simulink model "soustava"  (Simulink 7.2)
settings: Solver=ode45  StartTime=0.0  StopTime=1  RelTol=1e-3
InitFcn:
  | init_soustava;
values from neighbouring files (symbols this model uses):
  I1 = eye(3)    [init_soustava.m]
  I2 = [(m2/4)*(r2^2 + (h2^2)/3 ) 0 0    [init_soustava.m]
  I3 = [(m3/4)*(r3^2 + (h3^2)/3 ) 0 0    [init_soustava.m]
  m = 1    [smykadlo_init.m]
  m1 = 2    [init_soustava.m]
  m2 = 1    [init_soustava.m]
  m3 = 1    [init_soustava.m]
  r2 = 2    [init_soustava.m]
  r3 = 0.5    [init_soustava.m]
  rr = r3 + r2    (= 2.5)    [init_soustava.m]
undefined symbols (not defined in the file or in its folder): deg, kg, N, rad, s
libraries: mblibv1 x25

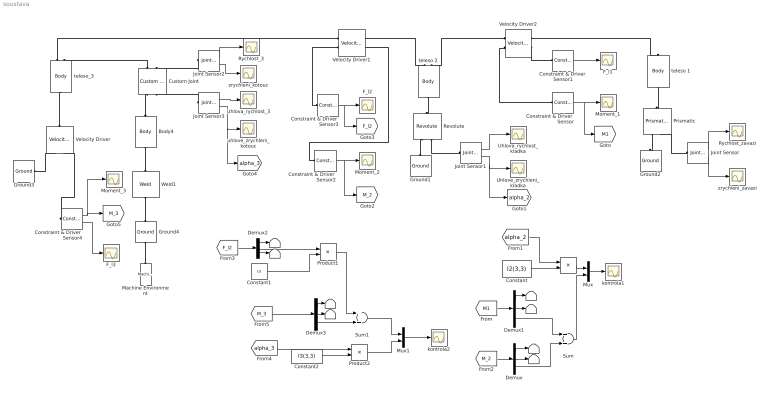
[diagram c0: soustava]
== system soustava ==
  " " : Terminator
  "   " : Terminator
  "       " : Terminator
  "        " : Terminator
  "         " : Terminator
  "          " : Terminator
  "           " : Terminator
  "               " : Product  OutDataType=sfix(16)  OutScaling=2^0
  "                  " : Terminator
  Body4 : mblibv1/Bodies/Body  Orientation=up  DialogController=MECH.DynMechDlgSource  PhysicalDomain=mechanical  SubClassName=Unknown  LeftPortType=workingframe  RightPortType=workingframe  LConnTagsString=CS1  RConnTagsString=CS2  UpdateFromCAD=off  DialogClass=MechanicalBodyBlock  Mass=0  MassUnits=kg  InertiaUnits=kg*m^2  Inertia=zeros(3)  Shape=Cylinder  ShapeDims=[1 1]  ShapeUnits=m  ShapeUse=false  Density=1  DensityUnits=kg/m^3  DensityUse=false  GraphicsMode=MACHINE_DEFAULT  BodyColorSelMode=MACHINE_DEFAULT  BodyColor=[1 0 0]  AttachedToCS=CG  CG=Left$CG$[0 0 0]$CS1$CS1$m$[0 0 0]$Euler X-Y-Z$deg$WORLD$false$none  WorkingFrames=Left$CS1$[0 0 0]$Adjoining$Adjoining$m$[0 0 0]$Euler X-Y-Z$deg$WORLD$true$none#Right$CS2$[0 0 0]$CS1$CS1$m$[0 0 0]$Euler X-Y-Z$deg$WORLD$true$none  CGPos=[0 0 0]  CGRot=[0 0 0]  CS0Pos=[]  CS0Rot=[]  CS1Pos=[0 0 0]  CS1Rot=[0 0 0]  CS2Pos=[0 0 0]  CS2Rot=[0 0 0]  CS3Pos=[]  CS3Rot=[]  CS4Pos=[]  CS4Rot=[]  CS5Pos=[]  CS5Rot=[]  CS6Pos=[]  CS6Rot=[]  CS7Pos=[]  CS7Rot=[]  CS8Pos=[]  CS8Rot=[]  CS9Pos=[]  CS9Rot=[]  CS10Pos=[]  CS10Rot=[]  CS11Pos=[]  CS11Rot=[]  CS12Pos=[]  CS12Rot=[]  CS13Pos=[]  CS13Rot=[]  CS14Pos=[]  CS14Rot=[]  CS15Pos=[]  CS15Rot=[]  CS16Pos=[]  CS16Rot=[]  CS17Pos=[]  CS17Rot=[]  CS18Pos=[]  CS18Rot=[]  CS19Pos=[]  CS19Rot=[]  CS20Pos=[]  CS20Rot=[]
  Constant : Constant  Value=I2(3,3)  OutDataType=sfix(16)  OutScaling=2^0
  Constant1 : Constant  Value=r3  OutDataType=sfix(16)  OutScaling=2^0
  Constant2 : Constant  Value=I3(3,3)  OutDataType=sfix(16)  OutScaling=2^0
  Constraint & Driver  Sensor : mblibv1/Sensors &  Actuators/Constraint & Driver  Sensor  DialogController=MECH.DynMechDlgSource  SystemSampleTime=-1  UpdateFromCAD=off  PhysicalDomain=Mechanical  DialogClass=ConstraintSensorBlock  SensedSide=Base  ReferenceFrame=Absolute (World)  ReactionForce=off  ForceUnits=N  ReactionMoment=on  MomentUnits=N*m  Muxed=on  OutputVector=[3 3]  ActiveIO=on  Width=3
  Constraint & Driver  Sensor1 : mblibv1/Sensors &  Actuators/Constraint & Driver  Sensor  DialogController=MECH.DynMechDlgSource  SystemSampleTime=-1  UpdateFromCAD=off  PhysicalDomain=Mechanical  DialogClass=ConstraintSensorBlock  SensedSide=Follower  ReferenceFrame=Absolute (World)  ReactionForce=on  ForceUnits=N  ReactionMoment=off  MomentUnits=N*m  Muxed=on  OutputVector=[3 3]  ActiveIO=on  Width=3
  Constraint & Driver  Sensor2 : mblibv1/Sensors &  Actuators/Constraint & Driver  Sensor  DialogController=MECH.DynMechDlgSource  SystemSampleTime=-1  UpdateFromCAD=off  PhysicalDomain=Mechanical  DialogClass=ConstraintSensorBlock  SensedSide=Follower  ReferenceFrame=Absolute (World)  ReactionForce=off  ForceUnits=N  ReactionMoment=on  MomentUnits=N*m  Muxed=on  OutputVector=[3 3]  ActiveIO=on  Width=3
  Constraint & Driver  Sensor3 : mblibv1/Sensors &  Actuators/Constraint & Driver  Sensor  DialogController=MECH.DynMechDlgSource  SystemSampleTime=-1  UpdateFromCAD=off  PhysicalDomain=Mechanical  DialogClass=ConstraintSensorBlock  SensedSide=Base  ReferenceFrame=Absolute (World)  ReactionForce=on  ForceUnits=N  ReactionMoment=off  MomentUnits=N*m  Muxed=on  OutputVector=[3 3]  ActiveIO=on  Width=3
  Constraint & Driver  Sensor4 : mblibv1/Sensors &  Actuators/Constraint & Driver  Sensor  DialogController=MECH.DynMechDlgSource  SystemSampleTime=-1  UpdateFromCAD=off  PhysicalDomain=Mechanical  DialogClass=ConstraintSensorBlock  SensedSide=Follower  ReferenceFrame=Absolute (World)  ReactionForce=on  ForceUnits=N  ReactionMoment=on  MomentUnits=N*m  Muxed=off  OutputVector=[3 3]  ActiveIO=on  Width=6
  Custom Joint : mblibv1/Joints/Custom Joint  Orientation=up  DialogController=MECH.DynMechDlgSource  PhysicalDomain=mechanical  SubClassName=custom_joint  LeftPortType=blob  RightPortType=blob  LConnTagsString=__newl0|SA1  RConnTagsString=__newr0|SA1  UpdateFromCAD=off  NumSAPorts=2  CutJoint=off  MarkAsCut=off  Primitives=prismatic  PrimitiveProps=P1$World$[0 1 0]$Prismatic#R1$World$[0 0 1]$Revolute  DialogClass=JointBlock  R1Axis=[0 0 1]  R2Axis=[]  R3Axis=[]  P1Axis=[0 1 0]  P2Axis=[]  P3Axis=[]  SAxis=[]
  Demux{,1..3} (4 alike) : Demux  Outputs=3
  F_l1 : Scope
  F_l2 : Scope
  F_l3 : Scope
  Ground1 : mblibv1/Bodies/Ground  Orientation=up  DialogController=MECH.DynMechDlgSource  SystemSampleTime=-1  UpdateFromCAD=off  LeftPortType=env  RightPortType=workingframe  PhysicalDomain=Mechanical  DialogClass=GroundBlock  CoordPosition=[0 0 0]  CoordPositionUnits=m  StateVectorMgrId=-1  MachineId=[0 0]  ShowEnvPort=off
  Ground2 : mblibv1/Bodies/Ground  Orientation=up  DialogController=MECH.DynMechDlgSource  SystemSampleTime=-1  UpdateFromCAD=off  LeftPortType=env  RightPortType=workingframe  PhysicalDomain=Mechanical  DialogClass=GroundBlock  CoordPosition=[r2 -1 0]  CoordPositionUnits=m  StateVectorMgrId=-1  MachineId=[0 0]  ShowEnvPort=off
  Ground3 : mblibv1/Bodies/Ground  DialogController=MECH.DynMechDlgSource  SystemSampleTime=-1  UpdateFromCAD=off  LeftPortType=env  RightPortType=workingframe  PhysicalDomain=Mechanical  DialogClass=GroundBlock  CoordPosition=[-(r3*2 + r2) 0 0]  CoordPositionUnits=m  StateVectorMgrId=-1  MachineId=[0 0]  ShowEnvPort=off
  Ground4 : mblibv1/Bodies/Ground  Orientation=up  DialogController=MECH.DynMechDlgSource  SystemSampleTime=-1  UpdateFromCAD=off  LeftPortType=env  RightPortType=workingframe  PhysicalDomain=Mechanical  DialogClass=GroundBlock  CoordPosition=[-rr 0 0]  CoordPositionUnits=m  StateVectorMgrId=-1  MachineId=[0 0]  ShowEnvPort=on
  Joint Sensor : mblibv1/Sensors &  Actuators/Joint Sensor  DialogController=MECH.DynMechDlgSource  SystemSampleTime=-1  UpdateFromCAD=off  PhysicalDomain=Mechanical  PortType=blob  Muxed=off  Pose=off  Angle=on  AngleUnits=deg  ArcVelocity=off  ArcVelocityUnits=deg/s  ArcAcceleration=off  ArcAccelerationUnits=deg/s^2  CoordPosition=off  CoordPositionUnits=m  Velocity=on  VelocityUnits=m/s  Acceleration=on  AccelerationUnits=m/s^2  Quaternion=on  QuaternionDT=off  QuaternionDDT=off  QuaternionUnits=off  OutputVector=[1]  ActiveIO=off  Width=2  DialogClass=MechanicalSensorBlock  Primitive=P1  Force=off  ForceUnits=N  Torque=off  TorqueUnits=N*m  ReferenceFrame=Absolute (World)  ReactionSensedSide=Base  ReactionReferenceFrame=Absolute (World)  ReactionForce=off  ReactionForceUnits=N  ReactionMoment=off  ReactionMomentUnits=N*m
  Joint Sensor1 : mblibv1/Sensors &  Actuators/Joint Sensor  DialogController=MECH.DynMechDlgSource  SystemSampleTime=-1  UpdateFromCAD=off  PhysicalDomain=Mechanical  PortType=blob  Muxed=off  Pose=off  Angle=off  AngleUnits=deg  ArcVelocity=on  ArcVelocityUnits=rad/s  ArcAcceleration=on  ArcAccelerationUnits=rad/s^2  CoordPosition=off  CoordPositionUnits=m  Velocity=on  VelocityUnits=m/s  Acceleration=off  AccelerationUnits=m/s^2  Quaternion=on  QuaternionDT=off  QuaternionDDT=off  QuaternionUnits=off  OutputVector=[1]  ActiveIO=off  Width=2  DialogClass=MechanicalSensorBlock  Primitive=R1  Force=off  ForceUnits=N  Torque=off  TorqueUnits=N*m  ReferenceFrame=Absolute (World)  ReactionSensedSide=Base  ReactionReferenceFrame=Absolute (World)  ReactionForce=off  ReactionForceUnits=N  ReactionMoment=off  ReactionMomentUnits=N*m
  Joint Sensor2 : mblibv1/Sensors &  Actuators/Joint Sensor  DialogController=MECH.DynMechDlgSource  SystemSampleTime=-1  UpdateFromCAD=off  PhysicalDomain=Mechanical  PortType=blob  Muxed=off  Pose=off  Angle=on  AngleUnits=deg  ArcVelocity=off  ArcVelocityUnits=deg/s  ArcAcceleration=off  ArcAccelerationUnits=deg/s^2  CoordPosition=off  CoordPositionUnits=m  Velocity=on  VelocityUnits=m/s  Acceleration=on  AccelerationUnits=m/s^2  Quaternion=on  QuaternionDT=off  QuaternionDDT=off  QuaternionUnits=off  OutputVector=[1]  ActiveIO=off  Width=2  DialogClass=MechanicalSensorBlock  Primitive=P1  Force=off  ForceUnits=N  Torque=off  TorqueUnits=N*m  ReferenceFrame=Absolute (World)  ReactionSensedSide=Base  ReactionReferenceFrame=Absolute (World)  ReactionForce=off  ReactionForceUnits=N  ReactionMoment=off  ReactionMomentUnits=N*m
  Joint Sensor3 : mblibv1/Sensors &  Actuators/Joint Sensor  DialogController=MECH.DynMechDlgSource  SystemSampleTime=-1  UpdateFromCAD=off  PhysicalDomain=Mechanical  PortType=blob  Muxed=off  Pose=off  Angle=off  AngleUnits=deg  ArcVelocity=on  ArcVelocityUnits=rad/s  ArcAcceleration=on  ArcAccelerationUnits=rad/s^2  CoordPosition=off  CoordPositionUnits=m  Velocity=on  VelocityUnits=m/s  Acceleration=off  AccelerationUnits=m/s^2  Quaternion=on  QuaternionDT=off  QuaternionDDT=off  QuaternionUnits=off  OutputVector=[1]  ActiveIO=off  Width=2  DialogClass=MechanicalSensorBlock  Primitive=R1  Force=off  ForceUnits=N  Torque=off  TorqueUnits=N*m  ReferenceFrame=Absolute (World)  ReactionSensedSide=Base  ReactionReferenceFrame=Absolute (World)  ReactionForce=off  ReactionForceUnits=N  ReactionMoment=off  ReactionMomentUnits=N*m
  Machine Environment : mblibv1/Bodies/Machine Environment  Orientation=up  DialogController=MECH.DialogSource  SystemSampleTime=-1  PortType=env  PhysicalDomain=Mechanical  DialogTemplateClass=MECH.MachineEnvironment  SyncWhenCopied=off  Gravity=[0 -9.81 0]  GravityUnits=m/s^2  GravityAsSignal=off  Dimensionality=Auto-detect  AnalysisType=Forward dynamics  LinearAssemblyTolerance=1e-3  LinearAssemblyToleranceUnits=m  AngularAssemblyTolerance=1e-3  AngularAssemblyToleranceUnits=rad  ConstraintSolverType=Stabilizing  ConstraintRelTolerance=1e-4  ConstraintAbsTolerance=1e-4  UseRobustSingularityHandling=off  RedundancyAnalysisToleranceType=Automatically select tolerance  RedundancyAnalysisTolerance=1e-14  StatePerturbationType=Fixed  PerturbationSize=1e-5  VisualizeMachine=on  BodyVisualizationType=Use model default body geometries  BodyColorSelMode=Use model default  DefaultBodyColor=[1 0 0]
  Moment_1 : Scope
  Moment_2 : Scope
  Moment_3 : Scope
  Mux : Mux  Inputs=2
  Mux1 : Mux  Inputs=2
  Prismatic : mblibv1/Joints/Prismatic  Orientation=up  DialogController=MECH.DynMechDlgSource  PhysicalDomain=mechanical  SubClassName=Unknown  LeftPortType=blob  RightPortType=blob  LConnTagsString=__newl0|SA1  RConnTagsString=__newr0  UpdateFromCAD=off  NumSAPorts=1  CutJoint=off  MarkAsCut=off  Primitives=prismatic  PrimitiveProps=P1$World$[0 1 0]$prismatic  DialogClass=JointBlock  P1Axis=[0 1 0]
  Product1 : Product  OutDataType=sfix(16)  OutScaling=2^0
  Product2 : Product  OutDataType=sfix(16)  OutScaling=2^0
  Revolute : mblibv1/Joints/Revolute  Orientation=up  DialogController=MECH.DynMechDlgSource  PhysicalDomain=mechanical  SubClassName=Unknown  LeftPortType=blob  RightPortType=blob  LConnTagsString=__newl0|SA1  RConnTagsString=__newr0  UpdateFromCAD=off  NumSAPorts=1  CutJoint=off  MarkAsCut=off  Primitives=prismatic  PrimitiveProps=R1$World$[0 0 1]$revolute  DialogClass=JointBlock  R1Axis=[0 0 1]
  Rychlost_3 : Scope
  Rychlost_zavazi : Scope
  Sum : Sum  OutDataType=sfix(16)  OutScaling=2^0
  Sum1 : Sum  OutDataType=sfix(16)  OutScaling=2^0
  Uhlova_rychlost_3 : Scope
  Uhlova_rychlost_kladka : Scope
  Uhlove_zrychleni_kladka : Scope
  Velocity Driver : mblibv1/Constraints &  Drivers/Velocity Driver  Orientation=up  DialogController=MECH.DynMechDlgSource  PhysicalDomain=mechanical  SubClassName=Unknown  LeftPortType=blob  RightPortType=blob  LConnTagsString=__newl0|SA1  RConnTagsString=__newr0  UpdateFromCAD=off  DialogClass=ConstantVelocityConstraint  NumSAPorts=1  Unit_V=m/s  Unit_Omega=rad/s  Coef_V_Base=[0 0 0]  Csys_V_Base=World  Coef_Omega_Base=[0 0 0]  Csys_Omega_Base=World  Coef_V_Follower=[0 1 0]  Csys_V_Follower=World  Coef_Omega_Follower=[0 0 -r3]  Csys_Omega_Follower=World
  Velocity Driver1 : mblibv1/Constraints &  Drivers/Velocity Driver  DialogController=MECH.DynMechDlgSource  PhysicalDomain=mechanical  SubClassName=Unknown  LeftPortType=blob  RightPortType=blob  LConnTagsString=__newl0|SA1  RConnTagsString=__newr0|SA1  UpdateFromCAD=off  DialogClass=ConstantVelocityConstraint  NumSAPorts=2  Unit_V=m/s  Unit_Omega=rad/s  Coef_V_Base=[0 1 0]  Csys_V_Base=World  Coef_Omega_Base=[0 0 r3]  Csys_Omega_Base=World  Coef_V_Follower=[0 0 0]  Csys_V_Follower=World  Coef_Omega_Follower=[0 0 -r2]  Csys_Omega_Follower=World
  Velocity Driver2 : mblibv1/Constraints &  Drivers/Velocity Driver  DialogController=MECH.DynMechDlgSource  PhysicalDomain=mechanical  SubClassName=Unknown  LeftPortType=blob  RightPortType=blob  LConnTagsString=__newl0|SA1  RConnTagsString=__newr0|SA1  UpdateFromCAD=off  DialogClass=ConstantVelocityConstraint  NumSAPorts=2  Unit_V=m/s  Unit_Omega=rad/s  Coef_V_Base=[0 0 0]  Csys_V_Base=World  Coef_Omega_Base=[0 0 r2]  Csys_Omega_Base=World  Coef_V_Follower=[0 1 0]  Csys_V_Follower=World  Coef_Omega_Follower=[0 0 0]  Csys_Omega_Follower=World
  Weld1 : mblibv1/Joints/Weld  Orientation=up  DialogController=MECH.DynMechDlgSource  PhysicalDomain=mechanical  SubClassName=Unknown  LeftPortType=blob  RightPortType=blob  LConnTagsString=__newl0  RConnTagsString=__newr0  UpdateFromCAD=off  NumSAPorts=0  CutJoint=off  MarkAsCut=off  Primitives=weld  PrimitiveProps=W$WORLD$[0 0 0]$weld  DialogClass=JointBlock  WAxis=[0 0 0]
  kontrola1 : Scope
  kontrola2 : Scope
  teleso 1 : mblibv1/Bodies/Body  Orientation=up  DialogController=MECH.DynMechDlgSource  PhysicalDomain=mechanical  SubClassName=Unknown  LeftPortType=workingframe  RightPortType=workingframe  LConnTagsString=CS1  RConnTagsString=CS2  UpdateFromCAD=off  DialogClass=MechanicalBodyBlock  Mass=m1  MassUnits=kg  InertiaUnits=kg*m^2  Inertia=I1  Shape=Cylinder  ShapeDims=[1 1]  ShapeUnits=m  ShapeUse=false  Density=1  DensityUnits=kg/m^3  DensityUse=false  GraphicsMode=MACHINE_DEFAULT  BodyColorSelMode=MACHINE_DEFAULT  BodyColor=[1 0 0]  AttachedToCS=CG  CG=Right$CG$[0 0 0]$CS1$CS1$m$[0 0 0]$Euler X-Y-Z$deg$WORLD$false$none  WorkingFrames=Left$CS1$[0 0 0]$Adjoining$Adjoining$m$[0 0 0]$Euler X-Y-Z$deg$WORLD$true$none#Right$CS2$[0 0 0]$CS1$CS1$m$[0 0 0]$Euler X-Y-Z$deg$WORLD$true$none  CGPos=[0 0 0]  CGRot=[0 0 0]  CS0Pos=[]  CS0Rot=[]  CS1Pos=[0 0 0]  CS1Rot=[0 0 0]  CS2Pos=[0 0 0]  CS2Rot=[0 0 0]  CS3Pos=[]  CS3Rot=[]  CS4Pos=[]  CS4Rot=[]  CS5Pos=[]  CS5Rot=[]  CS6Pos=[]  CS6Rot=[]  CS7Pos=[]  CS7Rot=[]  CS8Pos=[]  CS8Rot=[]  CS9Pos=[]  CS9Rot=[]  CS10Pos=[]  CS10Rot=[]  CS11Pos=[]  CS11Rot=[]  CS12Pos=[]  CS12Rot=[]  CS13Pos=[]  CS13Rot=[]  CS14Pos=[]  CS14Rot=[]  CS15Pos=[]  CS15Rot=[]  CS16Pos=[]  CS16Rot=[]  CS17Pos=[]  CS17Rot=[]  CS18Pos=[]  CS18Rot=[]  CS19Pos=[]  CS19Rot=[]  CS20Pos=[]  CS20Rot=[]
  teleso 2 : mblibv1/Bodies/Body  Orientation=up  DialogController=MECH.DynMechDlgSource  PhysicalDomain=mechanical  SubClassName=Unknown  LeftPortType=workingframe  RightPortType=workingframe  LConnTagsString=CG  RConnTagsString=CS2|CS1  UpdateFromCAD=off  DialogClass=MechanicalBodyBlock  Mass=m2  MassUnits=kg  InertiaUnits=kg*m^2  Inertia=I2  Shape=Cylinder  ShapeDims=[1 1]  ShapeUnits=m  ShapeUse=false  Density=1  DensityUnits=kg/m^3  DensityUse=false  GraphicsMode=MACHINE_DEFAULT  BodyColorSelMode=MACHINE_DEFAULT  BodyColor=[1 0 0]  AttachedToCS=CG  CG=Left$CG$[0 0 0]$Adjoining$Adjoining$m$[0 0 0]$Euler X-Y-Z$deg$WORLD$true$none  WorkingFrames=Right$CS2$[0 0 0]$CG$CG$m$[0 0 0]$Euler X-Y-Z$deg$WORLD$true$none#Right$CS1$[0 0 0]$CG$CG$m$[0 0 0]$Euler X-Y-Z$deg$WORLD$true$none  CGPos=[0 0 0]  CGRot=[0 0 0]  CS0Pos=[]  CS0Rot=[]  CS1Pos=[0 0 0]  CS1Rot=[0 0 0]  CS2Pos=[0 0 0]  CS2Rot=[0 0 0]  CS3Pos=[]  CS3Rot=[]  CS4Pos=[]  CS4Rot=[]  CS5Pos=[]  CS5Rot=[]  CS6Pos=[]  CS6Rot=[]  CS7Pos=[]  CS7Rot=[]  CS8Pos=[]  CS8Rot=[]  CS9Pos=[]  CS9Rot=[]  CS10Pos=[]  CS10Rot=[]  CS11Pos=[]  CS11Rot=[]  CS12Pos=[]  CS12Rot=[]  CS13Pos=[]  CS13Rot=[]  CS14Pos=[]  CS14Rot=[]  CS15Pos=[]  CS15Rot=[]  CS16Pos=[]  CS16Rot=[]  CS17Pos=[]  CS17Rot=[]  CS18Pos=[]  CS18Rot=[]  CS19Pos=[]  CS19Rot=[]  CS20Pos=[]  CS20Rot=[]
  teleso_3 : mblibv1/Bodies/Body  Orientation=down  DialogController=MECH.DynMechDlgSource  PhysicalDomain=mechanical  SubClassName=Unknown  LeftPortType=workingframe  RightPortType=workingframe  LConnTagsString=CG|CS1  RConnTagsString=CS2  UpdateFromCAD=off  DialogClass=MechanicalBodyBlock  Mass=m3  MassUnits=kg  InertiaUnits=kg*m^2  Inertia=I3  Shape=Cylinder  ShapeDims=[1 1]  ShapeUnits=m  ShapeUse=false  Density=1  DensityUnits=kg/m^3  DensityUse=false  GraphicsMode=MACHINE_DEFAULT  BodyColorSelMode=MACHINE_DEFAULT  BodyColor=[1 0 0]  AttachedToCS=CG  CG=Left$CG$[0 0 0]$CS1$CS1$m$[0 0 0]$Euler X-Y-Z$deg$WORLD$true$none  WorkingFrames=Right$CS2$[0 0 0]$CS1$CS1$m$[0 0 0]$Euler X-Y-Z$deg$WORLD$true$none#Left$CS1$[0 0 0]$Adjoining$Adjoining$m$[0 0 0]$Euler X-Y-Z$deg$WORLD$true$none  CGPos=[0 0 0]  CGRot=[0 0 0]  CS0Pos=[]  CS0Rot=[]  CS1Pos=[0 0 0]  CS1Rot=[0 0 0]  CS2Pos=[0 0 0]  CS2Rot=[0 0 0]  CS3Pos=[]  CS3Rot=[]  CS4Pos=[]  CS4Rot=[]  CS5Pos=[]  CS5Rot=[]  CS6Pos=[]  CS6Rot=[]  CS7Pos=[]  CS7Rot=[]  CS8Pos=[]  CS8Rot=[]  CS9Pos=[]  CS9Rot=[]  CS10Pos=[]  CS10Rot=[]  CS11Pos=[]  CS11Rot=[]  CS12Pos=[]  CS12Rot=[]  CS13Pos=[]  CS13Rot=[]  CS14Pos=[]  CS14Rot=[]  CS15Pos=[]  CS15Rot=[]  CS16Pos=[]  CS16Rot=[]  CS17Pos=[]  CS17Rot=[]  CS18Pos=[]  CS18Rot=[]  CS19Pos=[]  CS19Rot=[]  CS20Pos=[]  CS20Rot=[]
  uhlove_zrychleni_kotouc : Scope
  zrychleni_kotouc : Scope
  zrychleni_zavazi : Scope
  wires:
  Joint Sensor/1 -> Rychlost_zavazi/1
  Constraint & Driver  Sensor/1 -> Moment_1/1, [M1]
  Constraint & Driver  Sensor2/1 -> Moment_2/1, [M_2]
  Constraint & Driver  Sensor1/1 -> F_l1/1
  Constraint & Driver  Sensor4/2 -> F_l3/1
  Joint Sensor2/1 -> Rychlost_3/1
  Joint Sensor3/1 -> Uhlova_rychlost_3/1
  "               "/1 -> Mux/1
  Sum/1 -> Mux/2
  Mux/1 -> kontrola1/1
  Demux1/3 -> Sum/1
  Demux/3 -> Sum/2
  Constant/1 -> "               "/2
  Demux1/1 -> "           "/1
  Demux1/2 -> "                  "/1
  Demux/1 -> " "/1
  Demux/2 -> "   "/1
  Joint Sensor1/1 -> Uhlova_rychlost_kladka/1
  Joint Sensor1/2 -> Uhlove_zrychleni_kladka/1, [alpha_2]
  Constraint & Driver  Sensor3/1 -> F_l2/1, [F_l2]
  Demux2/2 -> Product1/1
  Demux2/1 -> "        "/1
  Demux2/3 -> "       "/1
  Constant1/1 -> Product1/2
  Product1/1 -> Sum1/1
  Demux3/1 -> "         "/1
  Demux3/2 -> "          "/1
  Demux3/3 -> Sum1/2
  Mux1/1 -> kontrola2/1
  Constant2/1 -> Product2/2
  Product2/1 -> Mux1/2
  Sum1/1 -> Mux1/1
  Joint Sensor2/2 -> zrychleni_kotouc/1
  Joint Sensor/2 -> zrychleni_zavazi/1
  Joint Sensor3/2 -> uhlove_zrychleni_kotouc/1, [alpha_3]
  Constraint & Driver  Sensor4/1 -> Moment_3/1, [M_3]
  [M1] -> Demux1/1
  [alpha_2] -> "               "/1
  [M_2] -> Demux/1
  [F_l2] -> Demux2/1
  [alpha_3] -> Product2/1
  [M_3] -> Demux3/1
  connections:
  Velocity Driver2/LConn1 -- teleso 2/RConn2
  Velocity Driver2/RConn1 -- teleso 1/RConn1
  Constraint & Driver  Sensor/LConn1 -- Velocity Driver2/LConn2
  Velocity Driver1/RConn1 -- teleso 2/RConn1
  Velocity Driver2/RConn2 -- Constraint & Driver  Sensor1/LConn1
  Constraint & Driver  Sensor3/LConn1 -- Velocity Driver1/LConn2
  Constraint & Driver  Sensor2/LConn1 -- Velocity Driver1/RConn2
  Body4/RConn1 -- Custom Joint/LConn1
  Weld1/RConn1 -- Body4/LConn1
  Ground3/RConn1 -- Velocity Driver/LConn1
  Custom Joint/RConn1 -- teleso_3/LConn2
  Velocity Driver/RConn1 -- teleso_3/RConn1
  Ground4/RConn1 -- Weld1/LConn1
  Constraint & Driver  Sensor4/LConn1 -- Velocity Driver/LConn2
  teleso_3/LConn1 -- Velocity Driver1/LConn1
  Machine Environment/RConn1 -- Ground4/LConn1
  Joint Sensor2/LConn1 -- Custom Joint/RConn2
  Joint Sensor3/LConn1 -- Custom Joint/LConn2
  teleso 2/LConn1 -- Revolute/RConn1
  Revolute/LConn2 -- Joint Sensor1/LConn1
  Ground1/RConn1 -- Revolute/LConn1
  teleso 1/LConn1 -- Prismatic/RConn1
  Joint Sensor/LConn1 -- Prismatic/LConn2
  Prismatic/LConn1 -- Ground2/RConn1
